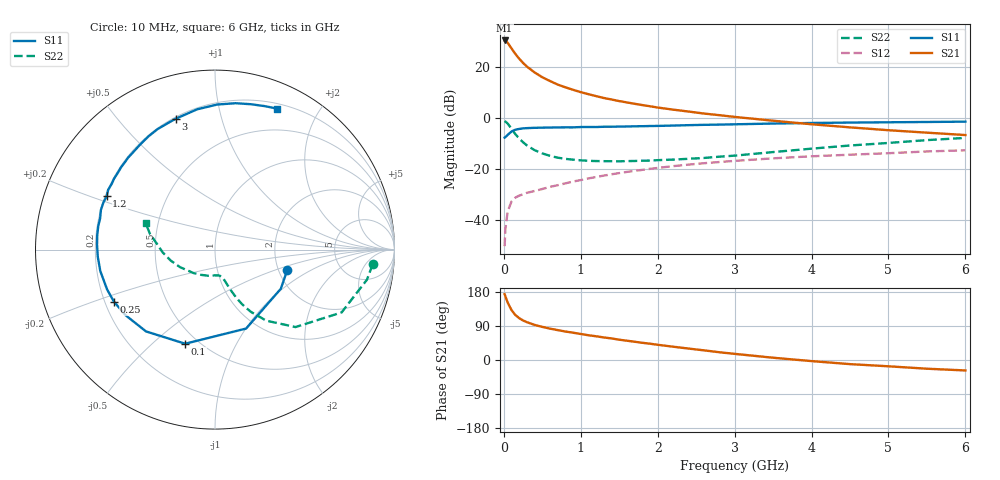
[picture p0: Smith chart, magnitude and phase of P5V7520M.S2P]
! SIEMENS Small Signal Semiconductors
! BFP183
! Si NPN RF Bipolar Junction Transistor in SOT143
! VCE = 0.75 V  IC = 20 mA
! Common Emitter S-Parameters:  March  1996
# GHz  S  MA  R  50
!  f  S11  S21  S12  S22
! GHz  MAG  ANG  MAG  ANG  MAG  ANG  MAG  ANG
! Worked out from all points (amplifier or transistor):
!   36 points, 10 MHz to 6 GHz, reference 50 ohm
!   highest |S21| = 30.5 dB at 10 MHz (marker M1)
!   |S21| within 3 dB of that: start of sweep to 96.9 MHz
!   unconditionally stable (mu >= 1): 461.8 MHz to end of sweep
!   at 250 MHz: K = 0.66, MSG = 25.8 dB, |S12| = -29.8 dB
!   at 1.4 GHz: K = 1.43, MAG = 10.8 dB, |S12| = -22.0 dB
!   at 6 GHz: K = 1.20, MAG = 0.3 dB, |S12| = -12.6 dB
!   S11 on the Smith chart (normalised r, x): 10 MHz: 2.24, -0.60; 100 MHz: 0.43, -0.64; 250 MHz: 0.24, -0.23; 1.2 GHz: 0.21, +0.22; 3 GHz: 0.21, +0.72; 6 GHz: 0.25, +1.50
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0.01  0.4184 -15.4  33.59 173.9  0.0031 80.8  0.882 -5.4
0.02  0.4268 -30.7  33.24 168.1  0.0067 76.8  0.8631 -11.2
0.05  0.4728 -68.5  30.19 151.4  0.0148 67.6  0.7875 -26.4
0.1  0.5502 -107.6  23.41 131.6  0.0234 51.7  0.6225 -43.9
0.15  0.5965 -130.2  18.24 118.7  0.0278 45.1  0.488 -54.2
0.2  0.6181 -143.8  14.71 110.4  0.0304 41.2  0.3994 -60.1
0.25  0.6334 -152.7  12.16 104.3  0.0323 40.3  0.3386 -63.7
0.3  0.6409 -159.8  10.32 99.8  0.0345 40.8  0.2929 -66.1
0.4  0.6501 -169.4  7.919 92.6  0.0375 41.8  0.2369 -69.2
0.5  0.6545 -176.6  6.377 87.4  0.041 43.0  0.2044 -70.9
0.6  0.6578 177.6  5.374 82.8  0.0452 45.4  0.1833 -72.5
0.7  0.6613 172.7  4.582 78.9  0.0486 46.9  0.1688 -74.0
0.9  0.6632 164.8  3.62 72.0  0.0575 49.0  0.154 -77.3
1.1  0.675 157.2  2.966 65.3  0.0661 49.9  0.1463 -81.2
1.2  0.6729 153.7  2.716 62.6  0.0704 49.9  0.1448 -83.3
1.6  0.69 141.7  2.047 50.9  0.0887 49.1  0.1445 -93.4
2.2  0.7191 125.3  1.477 35.1  0.1149 44.8  0.1546 -112.4
3  0.7611 106.8  1.064 16.2  0.1459 37.5  0.1849 -138.6
3.5  0.7881 97.2  0.895 6.0  0.1637 32.8  0.2173 -153.1
4.5  0.8236 82.0  0.663 -10.9  0.193 23.0  0.2923 -177.0
5.5  0.8457 71.0  0.522 -23.0  0.2235 14.6  0.373 166.4
6  0.8585 66.2  0.469 -27.6  0.2353 9.7  0.4121 159.3
